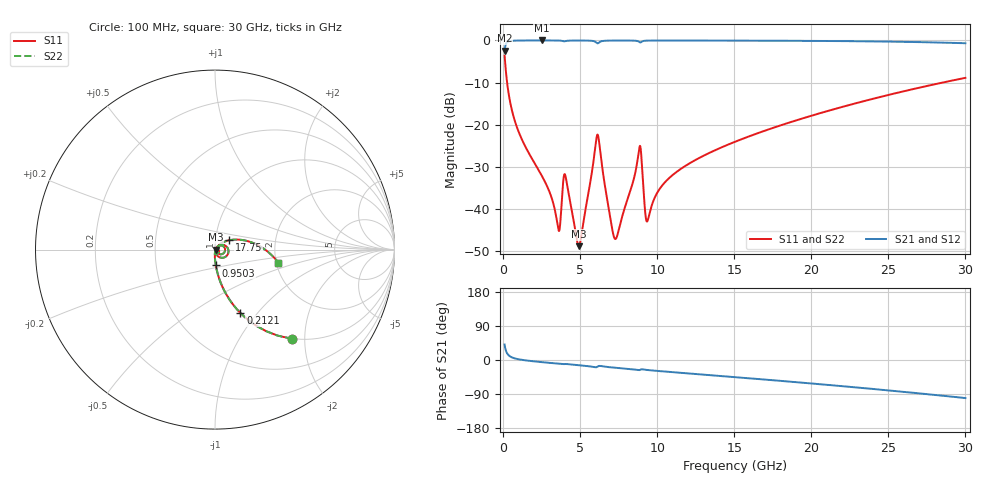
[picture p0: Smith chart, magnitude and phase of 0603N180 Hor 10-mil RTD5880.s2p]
# GHz S MA R 50
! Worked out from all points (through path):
!   3201 points, 100 MHz to 30 GHz, reference 50 ohm
!   highest |S21| = -0.02 dB at 2.52 GHz (marker M1); lowest = -2.5 dB at 100 MHz (marker M2)
!   group delay of S21, straight-line fit = 9.51 ps
!   lowest |S11| = -48.7 dB at 4.912 GHz (marker M3), VSWR 1.01, Z = 50.4 - j0.0933 ohm
!   |S11| at or under -10 dB: 261.5 MHz to 28.51 GHz (28.25 GHz wide, 196 % of centre)
!   |S22| runs from -48.7 to -3.6 dB; largest |S21 - S12| = 0
!   S11 on the Smith chart (normalised r, x): 100 MHz: 0.99, -1.74; 212.1 MHz: 0.99, -0.82; 950.3 MHz: 0.99, -0.18; 17.75 GHz: 1.17, +0.12; 30 GHz: 2.05, -0.34
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0.1  0.658 -49.1  0.7527 40.9  0.7527 40.9  0.658 -49.1
0.212125  0.3804 -68.2  0.9244 21.8  0.9244 21.8  0.3804 -68.2
0.5017812  0.1699 -81.4  0.9848 8.4  0.9848 8.4  0.1699 -81.4
0.9502812  0.08829 -87.0  0.9952 2.4  0.9952 2.4  0.08829 -87.0
2.520031  0.02479 -92.2  0.9982 -5.7  0.9982 -5.7  0.02479 -92.2
3.585219  0.005786 -54.7  0.9958 -9.9  0.9958 -9.9  0.005786 -54.7
3.930938  0.02368 -16.2  0.9764 -10.9  0.9764 -10.9  0.02368 -16.2
4.06175  0.02418 -52.2  0.9817 -10.5  0.9817 -10.5  0.02418 -52.2
4.912031  0.003652 -14.7  0.9963 -13.8  0.9963 -13.8  0.003652 -14.7
5.089563  0.004965 25.7  0.9961 -14.5  0.9961 -14.5  0.004965 25.7
6.117375  0.07637 -9.0  0.9244 -17.9  0.9244 -17.9  0.07637 -9.0
7.257313  0.004455 -19.3  0.9954 -20.4  0.9954 -20.4  0.004455 -19.3
8.836406  0.0528 15.0  0.9599 -26.7  0.9599 -26.7  0.0528 15.0
8.967219  0.04365 -36.8  0.9572 -24.5  0.9572 -24.5  0.04365 -36.8
9.200812  0.01021 -41.8  0.9901 -25.6  0.9901 -25.6  0.01021 -41.8
9.331625  0.007148 -4.6  0.9932 -26.2  0.9932 -26.2  0.007148 -4.6
10.06978  0.01644 47.6  0.9959 -29.0  0.9959 -29.0  0.01644 47.6
15.05  0.06296 41.2  0.9938 -45.2  0.9938 -45.2  0.06296 41.2
17.75034  0.09504 33.2  0.9908 -54.2  0.9908 -54.2  0.09504 33.2
20.03956  0.1286 25.8  0.9865 -62.0  0.9865 -62.0  0.1286 25.8
25.01978  0.2262 8.2  0.9677 -80.3  0.9677 -80.3  0.2262 8.2
30  0.3599 -11.6  0.9252 -100.4  0.9252 -100.4  0.3599 -11.6
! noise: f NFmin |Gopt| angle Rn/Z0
0.1  0.0003072  0.9224  0.4458  0.0008758
3.417  0.004521  0.8286  9.63  0.005513
6.743  0.01034  0.8511  18.93  0.0144
10.06  0.009122  0.762  28.05  0.007326
13.39  0.01044  0.7308  36.99  0.006967
16.7  0.01242  0.7224  45.7  0.007567
20.03  0.01454  0.7197  54.21  0.008193
23.35  0.0168  0.7209  62.45  0.008807
26.67  0.01927  0.7253  70.46  0.009413
30  0.022  0.7322  78.23  0.01002
